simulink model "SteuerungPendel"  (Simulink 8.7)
settings: Solver=ode45  StartTime=0.0  StopTime=T+1  MaxStep=1e-2  RelTol=1e-6

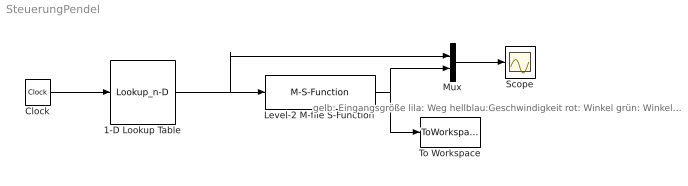
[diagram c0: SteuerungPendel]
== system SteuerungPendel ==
  note: gelb: Eingangsgröße lila: Weg hellblau:Geschwindigkeit rot: Winkel grün: Winkelgeschwindigkeit
  1-D Lookup Table : Lookup_n-D  NumberOfTableDimensions=1  BreakpointsForDimension1=t  Table=u  ExtrapMethod=Clip  UseLastTableValue=on  InternalRulePriority=Speed  RndMeth=Simplest
  Clock : Clock
  Level-2 M-file S-Function : M-S-Function  FunctionName=systemPendel_V5  Parameters=stPendel, x0
  Mux : Mux  Inputs=2
  Scope : Scope
  To Workspace : ToWorkspace  VariableName=mStates  SampleTime=-1
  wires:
  Level-2 M-file S-Function/1 -> To Workspace/1, Mux/2
  Clock/1 -> 1-D Lookup Table/1
  Mux/1 -> Scope/1
  1-D Lookup Table/1 -> Mux/1, Level-2 M-file S-Function/1
